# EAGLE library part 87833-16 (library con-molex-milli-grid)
HEADER
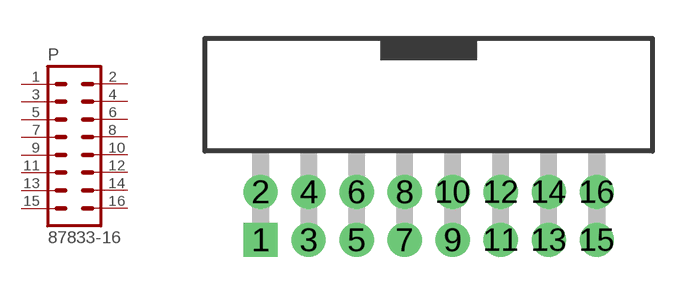
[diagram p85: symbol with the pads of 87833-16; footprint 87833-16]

Designator prefix P

## 87833-16  [87833-16]
1  1  pas
2  2  pas
3  3  pas
4  4  pas
5  5  pas
6  6  pas
7  7  pas
8  8  pas
9  9  pas
10  10  pas
11  11  pas
12  12  pas
13  13  pas
14  14  pas
15  15  pas
16  16  pas

## Footprint 87833-16 (pad centres in mm)
HEADER Dual Row, Shrouded, Right Angle
drill 0.914 square: 1 -7,-1
drill 0.914: 2 -7,1; 3 -5,-1; 4 -5,1; 5 -3,-1; 6 -3,1; 7 -1,-1; 8 -1,1; 9 1,-1; 10 1,1; 11 3,-1; 12 3,1; 13 5,-1; 14 5,1; 15 7,-1; 16 7,1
